(* Logix 5000 AddOnInstructionDefinition export Banner_QM30VT3_PD_v5; software revision 33.00 *)

TYPE Banner_QM30VT3_FP_RMS_PD_v5 :
STRUCT
   X_RMS_Velocity : REAL;   // in/sec or mm/sec
   Y_RMS_Velocity : REAL;   // in/sec or mm/sec
   Z_RMS_Velocity : REAL;   // in/sec or mm/sec
   X_High_Freq_RMS_Accel : REAL;   // G
   Y_High_Freq_RMS_Accel : REAL;   // G
   Z_High_Freq_RMS_Accel : REAL;   // G
   Temperature : REAL;   // F or C
   X : Banner_QM30VT3_FP_RMS_XYZ_PD_v5;
   Y : Banner_QM30VT3_FP_RMS_XYZ_PD_v5;
   Z : Banner_QM30VT3_FP_RMS_XYZ_PD_v5;
   Temp_Warning : BOOL;
   Temp_Alarm : BOOL;
END_STRUCT
END_TYPE

TYPE Banner_QM30VT3_FP_RMS_XYZ_PD_v5 :
STRUCT
   Vel_Acute_Warning : BOOL;
   Vel_Acute_Alarm : BOOL;
   Vel_Chronic_Warning : BOOL;
   Vel_Chronic_Alarm : BOOL;
   HiFreq_Accel_Acute_Warning : BOOL;
   HiFreq_Accel_Acute_Alarm : BOOL;
   HiFreq_Accel_Chronic_Warning : BOOL;
   HiFreq_Accel_Chronic_Alarm : BOOL;
END_STRUCT
END_TYPE

TYPE Banner_QM30VT3_PDI_v5 :
STRUCT
   PD0_FP_imperial : Banner_QM30VT3_FP_RMS_PD_v5;
   PD1_SS_imperial : Banner_QM30VT3_SS_RMS_PD_v5;
   PD2_FP_metric : Banner_QM30VT3_FP_RMS_PD_v5;
   PD3_SS_metric : Banner_QM30VT3_SS_RMS_PD_v5;
   PD4_User_metric : Banner_QM30VT3_User_PD_v5;
   PD5_User_imperial : Banner_QM30VT3_User_PD_v5;
   DTI : SINT[32];
END_STRUCT
END_TYPE

TYPE Banner_QM30VT3_SS_RMS_PD_HiFreq_v5 :
STRUCT
   High_Frequency_RMS_Accel : DINT;
   Scale : INT;
   HiFreq_Accel_Acute_Warning : BOOL;
   HiFreq_Accel_Acute_Alarm : BOOL;
   HiFreq_Accel_Chronic_Warning : BOOL;
   HiFreq_Accel_Chronice_Alarm : BOOL;
END_STRUCT
END_TYPE

TYPE Banner_QM30VT3_SS_RMS_PD_v5 :
STRUCT
   X_Velocity : Banner_QM30VT3_SS_RMS_Vel_PD_v5;
   Y_Velocity : Banner_QM30VT3_SS_RMS_Vel_PD_v5;
   Z_Velocity : Banner_QM30VT3_SS_RMS_Vel_PD_v5;
   X_HiFreq : Banner_QM30VT3_SS_RMS_PD_HiFreq_v5;
   Y_HiFreq : Banner_QM30VT3_SS_RMS_PD_HiFreq_v5;
   Z_HiFreq : Banner_QM30VT3_SS_RMS_PD_HiFreq_v5;
   Temperature : DINT;   // F or C
   Scale : INT;
   Temp_Warning : BOOL;
   Temp_Alarm : BOOL;
END_STRUCT
END_TYPE

TYPE Banner_QM30VT3_SS_RMS_Vel_PD_v5 :
STRUCT
   RMS_Velocity : DINT;   // in/s or mm/sec
   Scale : INT;
   Vel_Acute_Warning : BOOL;
   Vel_Acute_Alarm : BOOL;
   Vel_Chronic_Warning : BOOL;
   Vel_Chronic_Alarm : BOOL;
END_STRUCT
END_TYPE

TYPE Banner_QM30VT3_User_PD_v5 :
STRUCT
   Metric : REAL[8];
   M1_Chan_1_Warning : BOOL;
   M1_Chan_2_Alarm : BOOL;
   M2_Chan_1_Warning : BOOL;
   M2_Chan_2_Alarm : BOOL;
   M3_Chan_1_Warning : BOOL;
   M3_Chan_2_Alarm : BOOL;
   M4_Chan_1_Warning : BOOL;
   M4_Chan_2_Alarm : BOOL;
   M5_Chan_1_Warning : BOOL;
   M5_Chan_2_Alarm : BOOL;
   M6_Chan_1_Warning : BOOL;
   M6_Chan_2_Alarm : BOOL;
   M7_Chan_1_Warning : BOOL;
   M7_Chan_2_Alarm : BOOL;
END_STRUCT
END_TYPE

ADD_ON_INSTRUCTION Banner_QM30VT3_PD_FP_RMS_v5   (* revision 1.0 *)
VAR_IN_OUT
   Bytes : SINT[32]; {required}
   Data : Banner_QM30VT3_FP_RMS_PD_v5; {required}
END_VAR
VAR
   Temp : DINT[16]; {access None}
END_VAR

ROUTINE Logic   (* ladder *)
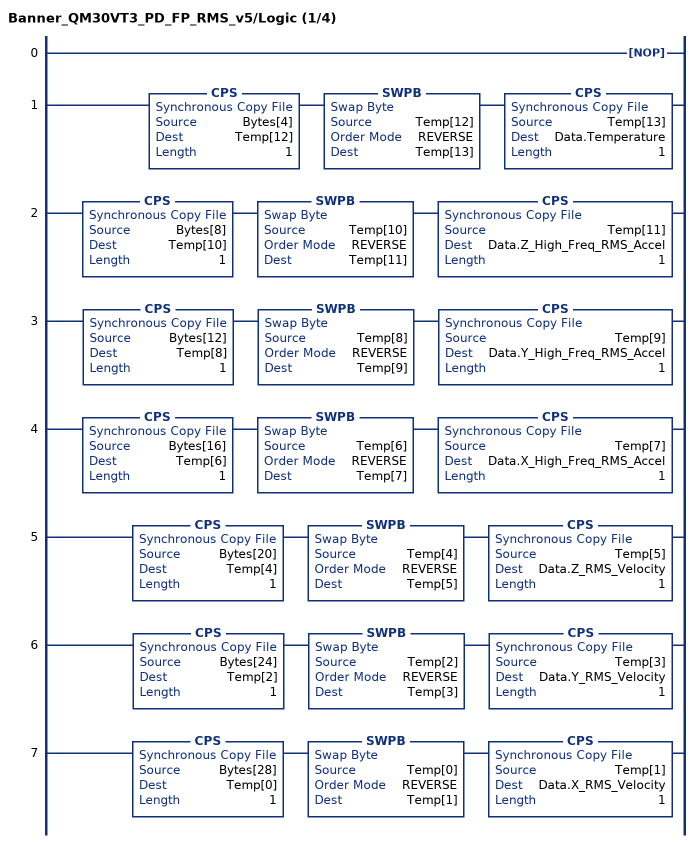
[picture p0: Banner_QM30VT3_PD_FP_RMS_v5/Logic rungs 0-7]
   0: NOP();
   1: CPS(Bytes[4],Temp[12],1)SWPB(Temp[12],REVERSE,Temp[13])CPS(Temp[13],Data.Temperature,1);
   2: CPS(Bytes[8],Temp[10],1)SWPB(Temp[10],REVERSE,Temp[11])CPS(Temp[11],Data.Z_High_Freq_RMS_Accel,1);
   3: CPS(Bytes[12],Temp[8],1)SWPB(Temp[8],REVERSE,Temp[9])CPS(Temp[9],Data.Y_High_Freq_RMS_Accel,1);
   4: CPS(Bytes[16],Temp[6],1)SWPB(Temp[6],REVERSE,Temp[7])CPS(Temp[7],Data.X_High_Freq_RMS_Accel,1);
   5: CPS(Bytes[20],Temp[4],1)SWPB(Temp[4],REVERSE,Temp[5])CPS(Temp[5],Data.Z_RMS_Velocity,1);
   6: CPS(Bytes[24],Temp[2],1)SWPB(Temp[2],REVERSE,Temp[3])CPS(Temp[3],Data.Y_RMS_Velocity,1);
   7: CPS(Bytes[28],Temp[0],1)SWPB(Temp[0],REVERSE,Temp[1])CPS(Temp[1],Data.X_RMS_Velocity,1);
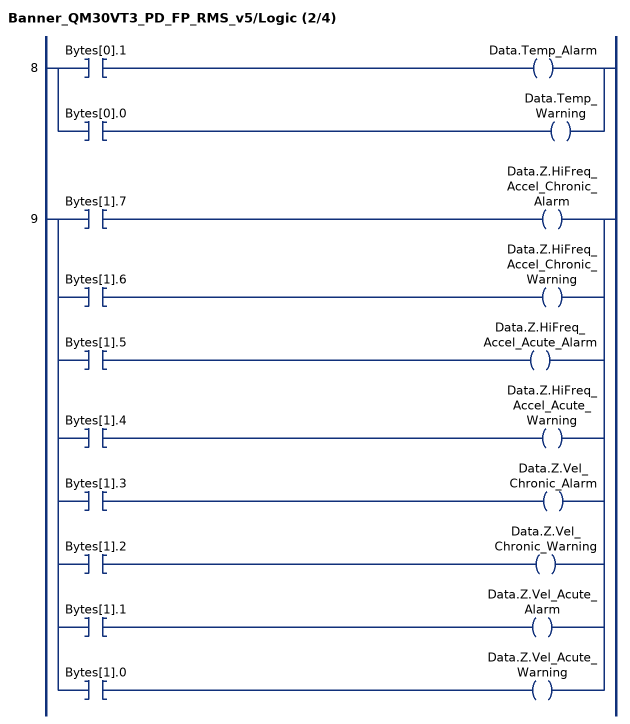
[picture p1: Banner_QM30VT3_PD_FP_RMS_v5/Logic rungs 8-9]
   8: [XIC(Bytes[0].1) OTE(Data.Temp_Alarm) ,XIC(Bytes[0].0) OTE(Data.Temp_Warning) ];
   9: [XIC(Bytes[1].7) OTE(Data.Z.HiFreq_Accel_Chronic_Alarm) ,XIC(Bytes[1].6) OTE(Data.Z.HiFreq_Accel_Chronic_Warning) ,XIC(Bytes[1].5) OTE(Data.Z.HiFreq_Accel_Acute_Alarm) ,XIC(Bytes[1].4) OTE(Data.Z.HiFreq_Accel_Acute_Warning) ,XIC(Bytes[1].3) OTE(Data.Z.Vel_Chronic_Alarm) ,XIC(Bytes[1].2) OTE(Data.Z.Vel_Chronic_Warning) ,XIC(Bytes[1].1) OTE(Data.Z.Vel_Acute_Alarm) ,XIC(Bytes[1].0) OTE(Data.Z.Vel_Acute_Warning) ];
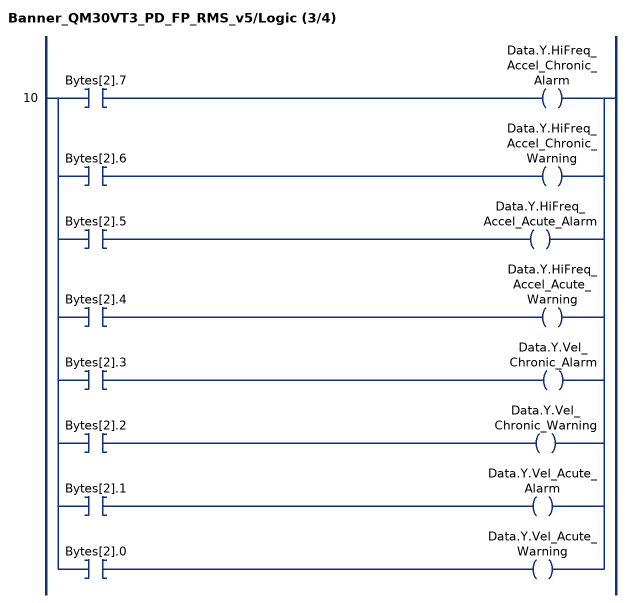
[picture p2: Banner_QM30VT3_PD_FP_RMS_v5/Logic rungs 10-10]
   10: [XIC(Bytes[2].7) OTE(Data.Y.HiFreq_Accel_Chronic_Alarm) ,XIC(Bytes[2].6) OTE(Data.Y.HiFreq_Accel_Chronic_Warning) ,XIC(Bytes[2].5) OTE(Data.Y.HiFreq_Accel_Acute_Alarm) ,XIC(Bytes[2].4) OTE(Data.Y.HiFreq_Accel_Acute_Warning) ,XIC(Bytes[2].3) OTE(Data.Y.Vel_Chronic_Alarm) ,XIC(Bytes[2].2) OTE(Data.Y.Vel_Chronic_Warning) ,XIC(Bytes[2].1) OTE(Data.Y.Vel_Acute_Alarm) ,XIC(Bytes[2].0) OTE(Data.Y.Vel_Acute_Warning) ];
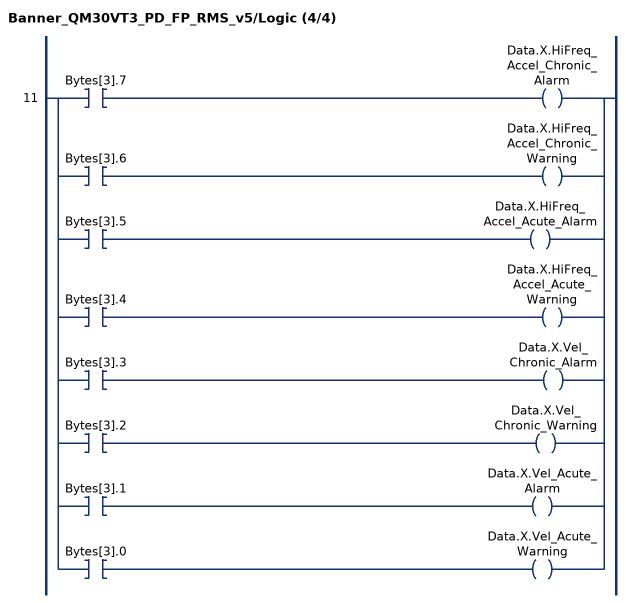
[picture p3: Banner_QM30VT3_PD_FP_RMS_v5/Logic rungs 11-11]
   11: [XIC(Bytes[3].7) OTE(Data.X.HiFreq_Accel_Chronic_Alarm) ,XIC(Bytes[3].6) OTE(Data.X.HiFreq_Accel_Chronic_Warning) ,XIC(Bytes[3].5) OTE(Data.X.HiFreq_Accel_Acute_Alarm) ,XIC(Bytes[3].4) OTE(Data.X.HiFreq_Accel_Acute_Warning) ,XIC(Bytes[3].3) OTE(Data.X.Vel_Chronic_Alarm) ,XIC(Bytes[3].2) OTE(Data.X.Vel_Chronic_Warning) ,XIC(Bytes[3].1) OTE(Data.X.Vel_Acute_Alarm) ,XIC(Bytes[3].0) OTE(Data.X.Vel_Acute_Warning) ];
END_ROUTINE
END_ADD_ON_INSTRUCTION

ADD_ON_INSTRUCTION Banner_QM30VT3_PD_SS_RMS_v5   (* revision 1.0 *)
VAR_IN_OUT
   Bytes : SINT[32]; {required}
   Data : Banner_QM30VT3_SS_RMS_PD_v5; {required}
END_VAR
VAR
   Temp : DINT[16]; {access None}
END_VAR

ROUTINE Logic   (* ladder *)
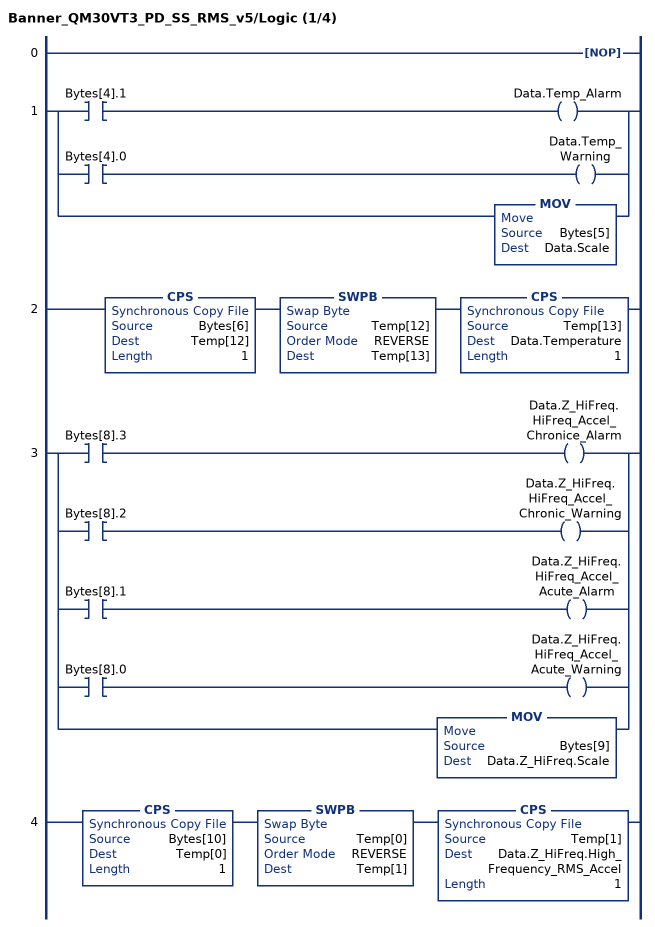
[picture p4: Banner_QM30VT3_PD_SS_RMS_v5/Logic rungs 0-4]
   0: NOP();
   1: [XIC(Bytes[4].1) OTE(Data.Temp_Alarm) ,XIC(Bytes[4].0) OTE(Data.Temp_Warning) ,MOV(Bytes[5],Data.Scale) ];
   2: CPS(Bytes[6],Temp[12],1)SWPB(Temp[12],REVERSE,Temp[13])CPS(Temp[13],Data.Temperature,1);
   3: [XIC(Bytes[8].3) OTE(Data.Z_HiFreq.HiFreq_Accel_Chronice_Alarm) ,XIC(Bytes[8].2) OTE(Data.Z_HiFreq.HiFreq_Accel_Chronic_Warning) ,XIC(Bytes[8].1) OTE(Data.Z_HiFreq.HiFreq_Accel_Acute_Alarm) ,XIC(Bytes[8].0) OTE(Data.Z_HiFreq.HiFreq_Accel_Acute_Warning) ,MOV(Bytes[9],Data.Z_HiFreq.Scale) ];
   4: CPS(Bytes[10],Temp[0],1)SWPB(Temp[0],REVERSE,Temp[1])CPS(Temp[1],Data.Z_HiFreq.High_Frequency_RMS_Accel,1);
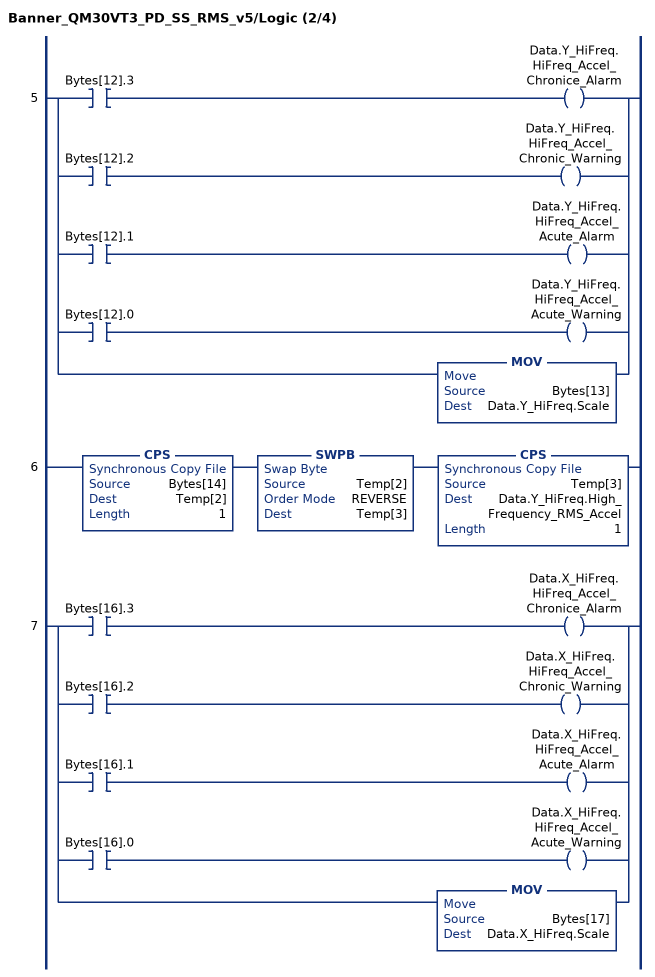
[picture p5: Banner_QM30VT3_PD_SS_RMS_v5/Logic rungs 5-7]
   5: [XIC(Bytes[12].3) OTE(Data.Y_HiFreq.HiFreq_Accel_Chronice_Alarm) ,XIC(Bytes[12].2) OTE(Data.Y_HiFreq.HiFreq_Accel_Chronic_Warning) ,XIC(Bytes[12].1) OTE(Data.Y_HiFreq.HiFreq_Accel_Acute_Alarm) ,XIC(Bytes[12].0) OTE(Data.Y_HiFreq.HiFreq_Accel_Acute_Warning) ,MOV(Bytes[13],Data.Y_HiFreq.Scale) ];
   6: CPS(Bytes[14],Temp[2],1)SWPB(Temp[2],REVERSE,Temp[3])CPS(Temp[3],Data.Y_HiFreq.High_Frequency_RMS_Accel,1);
   7: [XIC(Bytes[16].3) OTE(Data.X_HiFreq.HiFreq_Accel_Chronice_Alarm) ,XIC(Bytes[16].2) OTE(Data.X_HiFreq.HiFreq_Accel_Chronic_Warning) ,XIC(Bytes[16].1) OTE(Data.X_HiFreq.HiFreq_Accel_Acute_Alarm) ,XIC(Bytes[16].0) OTE(Data.X_HiFreq.HiFreq_Accel_Acute_Warning) ,MOV(Bytes[17],Data.X_HiFreq.Scale) ];
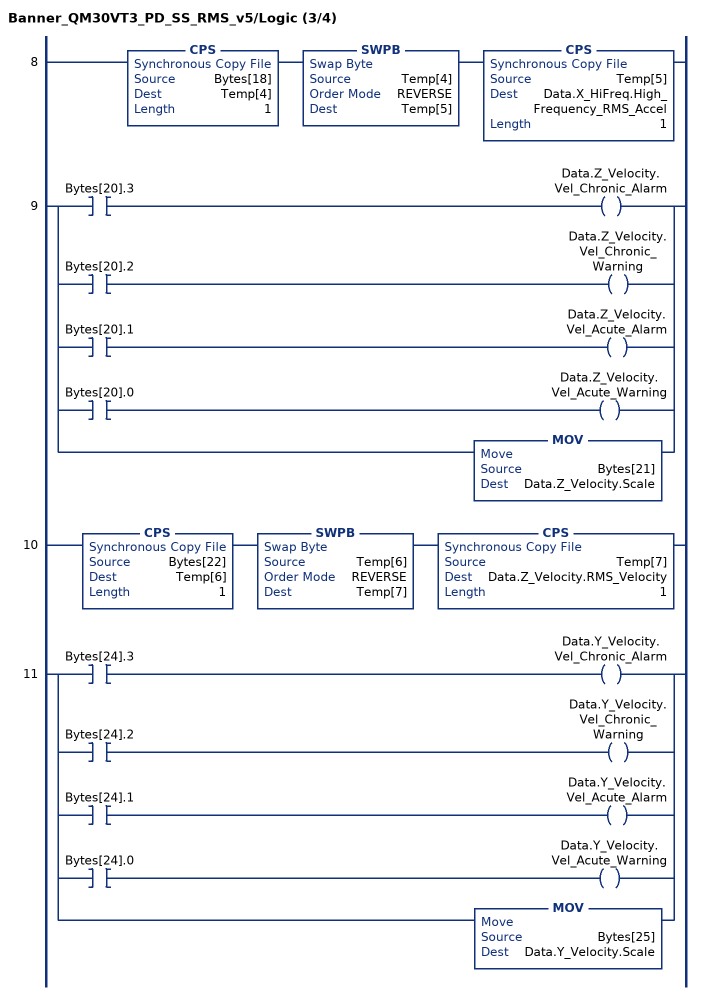
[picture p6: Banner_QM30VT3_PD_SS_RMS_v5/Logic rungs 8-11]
   8: CPS(Bytes[18],Temp[4],1)SWPB(Temp[4],REVERSE,Temp[5])CPS(Temp[5],Data.X_HiFreq.High_Frequency_RMS_Accel,1);
   9: [XIC(Bytes[20].3) OTE(Data.Z_Velocity.Vel_Chronic_Alarm) ,XIC(Bytes[20].2) OTE(Data.Z_Velocity.Vel_Chronic_Warning) ,XIC(Bytes[20].1) OTE(Data.Z_Velocity.Vel_Acute_Alarm) ,XIC(Bytes[20].0) OTE(Data.Z_Velocity.Vel_Acute_Warning) ,MOV(Bytes[21],Data.Z_Velocity.Scale) ];
   10: CPS(Bytes[22],Temp[6],1)SWPB(Temp[6],REVERSE,Temp[7])CPS(Temp[7],Data.Z_Velocity.RMS_Velocity,1);
   11: [XIC(Bytes[24].3) OTE(Data.Y_Velocity.Vel_Chronic_Alarm) ,XIC(Bytes[24].2) OTE(Data.Y_Velocity.Vel_Chronic_Warning) ,XIC(Bytes[24].1) OTE(Data.Y_Velocity.Vel_Acute_Alarm) ,XIC(Bytes[24].0) OTE(Data.Y_Velocity.Vel_Acute_Warning) ,MOV(Bytes[25],Data.Y_Velocity.Scale) ];
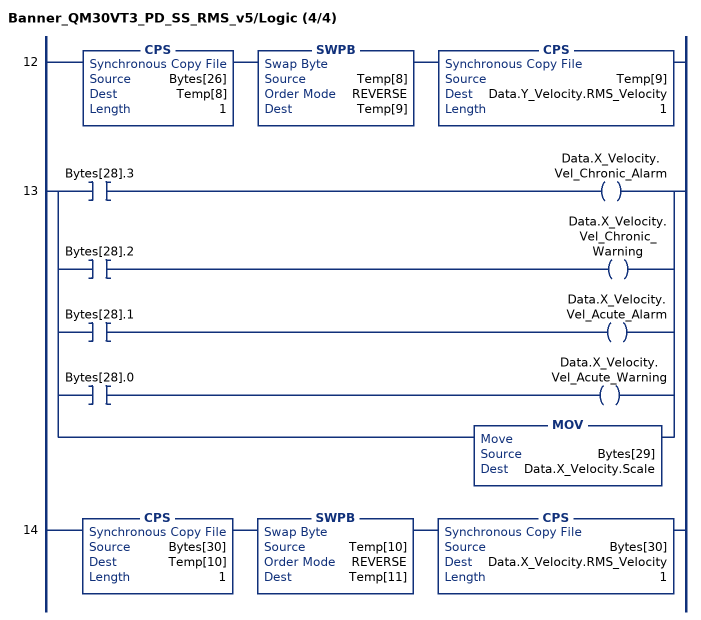
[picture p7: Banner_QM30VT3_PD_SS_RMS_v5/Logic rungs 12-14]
   12: CPS(Bytes[26],Temp[8],1)SWPB(Temp[8],REVERSE,Temp[9])CPS(Temp[9],Data.Y_Velocity.RMS_Velocity,1);
   13: [XIC(Bytes[28].3) OTE(Data.X_Velocity.Vel_Chronic_Alarm) ,XIC(Bytes[28].2) OTE(Data.X_Velocity.Vel_Chronic_Warning) ,XIC(Bytes[28].1) OTE(Data.X_Velocity.Vel_Acute_Alarm) ,XIC(Bytes[28].0) OTE(Data.X_Velocity.Vel_Acute_Warning) ,MOV(Bytes[29],Data.X_Velocity.Scale) ];
   14: CPS(Bytes[30],Temp[10],1)SWPB(Temp[10],REVERSE,Temp[11])CPS(Bytes[30],Data.X_Velocity.RMS_Velocity,1);
END_ROUTINE
END_ADD_ON_INSTRUCTION

ADD_ON_INSTRUCTION Banner_QM30VT3_PD_User_v5   (* revision 1.0 *)
VAR_IN_OUT
   Bytes : SINT[32]; {required}
   Data : Banner_QM30VT3_User_PD_v5; {required}
END_VAR
VAR
   Temp : DINT[16]; {access None}
END_VAR

ROUTINE Logic   (* ladder *)
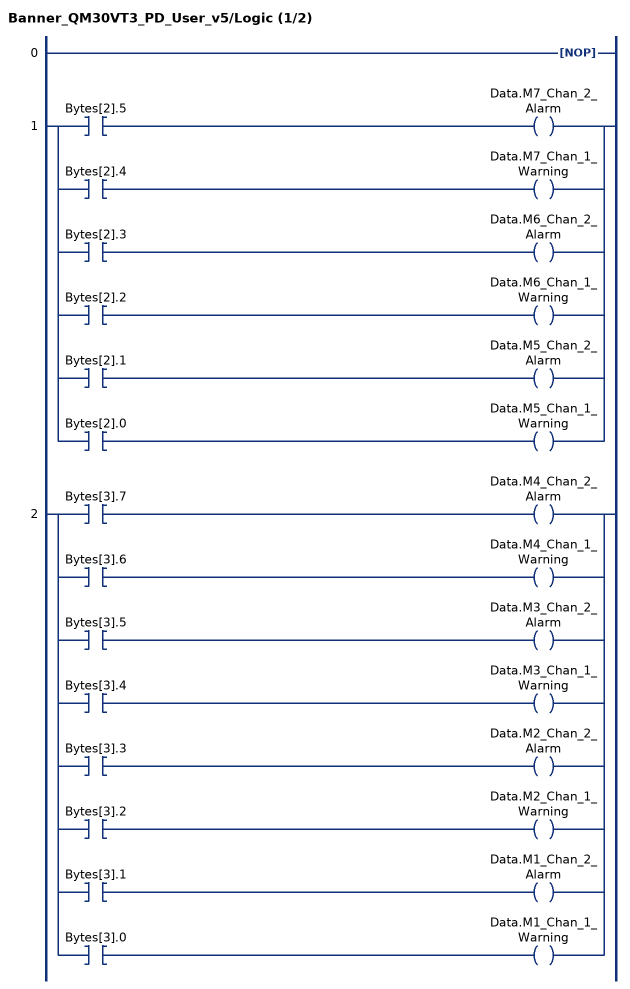
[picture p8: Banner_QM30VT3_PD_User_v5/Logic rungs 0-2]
   0: NOP();
   1: [XIC(Bytes[2].5) OTE(Data.M7_Chan_2_Alarm) ,XIC(Bytes[2].4) OTE(Data.M7_Chan_1_Warning) ,XIC(Bytes[2].3) OTE(Data.M6_Chan_2_Alarm) ,XIC(Bytes[2].2) OTE(Data.M6_Chan_1_Warning) ,XIC(Bytes[2].1) OTE(Data.M5_Chan_2_Alarm) ,XIC(Bytes[2].0) OTE(Data.M5_Chan_1_Warning) ];
   2: [XIC(Bytes[3].7) OTE(Data.M4_Chan_2_Alarm) ,XIC(Bytes[3].6) OTE(Data.M4_Chan_1_Warning) ,XIC(Bytes[3].5) OTE(Data.M3_Chan_2_Alarm) ,XIC(Bytes[3].4) OTE(Data.M3_Chan_1_Warning) ,XIC(Bytes[3].3) OTE(Data.M2_Chan_2_Alarm) ,XIC(Bytes[3].2) OTE(Data.M2_Chan_1_Warning) ,XIC(Bytes[3].1) OTE(Data.M1_Chan_2_Alarm) ,XIC(Bytes[3].0) OTE(Data.M1_Chan_1_Warning) ];
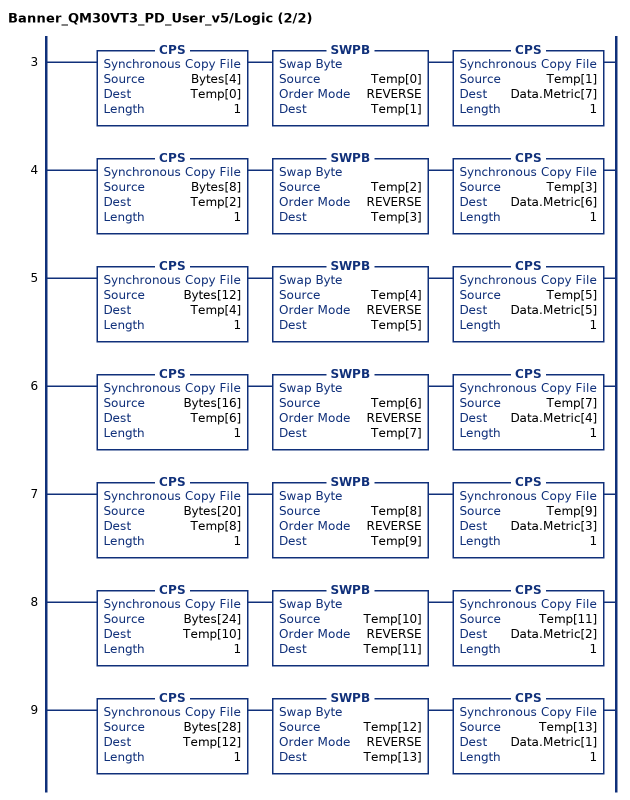
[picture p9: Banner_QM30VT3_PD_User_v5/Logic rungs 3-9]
   3: CPS(Bytes[4],Temp[0],1)SWPB(Temp[0],REVERSE,Temp[1])CPS(Temp[1],Data.Metric[7],1);
   4: CPS(Bytes[8],Temp[2],1)SWPB(Temp[2],REVERSE,Temp[3])CPS(Temp[3],Data.Metric[6],1);
   5: CPS(Bytes[12],Temp[4],1)SWPB(Temp[4],REVERSE,Temp[5])CPS(Temp[5],Data.Metric[5],1);
   6: CPS(Bytes[16],Temp[6],1)SWPB(Temp[6],REVERSE,Temp[7])CPS(Temp[7],Data.Metric[4],1);
   7: CPS(Bytes[20],Temp[8],1)SWPB(Temp[8],REVERSE,Temp[9])CPS(Temp[9],Data.Metric[3],1);
   8: CPS(Bytes[24],Temp[10],1)SWPB(Temp[10],REVERSE,Temp[11])CPS(Temp[11],Data.Metric[2],1);
   9: CPS(Bytes[28],Temp[12],1)SWPB(Temp[12],REVERSE,Temp[13])CPS(Temp[13],Data.Metric[1],1);
END_ROUTINE
END_ADD_ON_INSTRUCTION

ADD_ON_INSTRUCTION Banner_QM30VT3_PD_v5   (* revision 5.0 *)
VAR_IN_OUT
   QM30VT3 : Banner_QM30VT3_PDI_v5; {required}
END_VAR
VAR_INPUT
   Configuration : DINT; {required}
   Byte_Swap : BOOL; {required}
END_VAR
VAR
   Status_FP_RMS : Banner_QM30VT3_PD_FP_RMS_v5[2]; {access None}
   Status_SS_RMS : Banner_QM30VT3_PD_SS_RMS_v5[2]; {access None}
   Status_User : Banner_QM30VT3_PD_User_v5[2]; {access None}
END_VAR

ROUTINE Logic   (* ladder *)
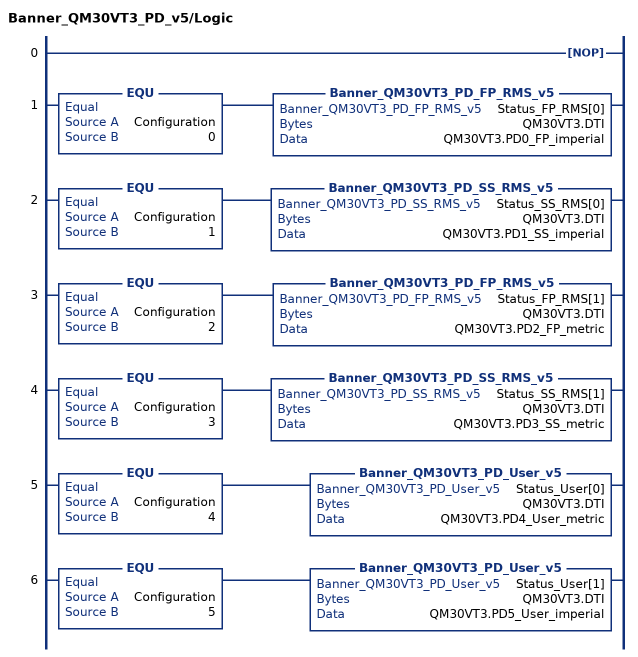
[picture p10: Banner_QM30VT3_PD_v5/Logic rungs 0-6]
   0: NOP();
   1: EQU(Configuration,0)Banner_QM30VT3_PD_FP_RMS_v5(Status_FP_RMS[0],QM30VT3.DTI,QM30VT3.PD0_FP_imperial);
   2: EQU(Configuration,1)Banner_QM30VT3_PD_SS_RMS_v5(Status_SS_RMS[0],QM30VT3.DTI,QM30VT3.PD1_SS_imperial);
   3: EQU(Configuration,2)Banner_QM30VT3_PD_FP_RMS_v5(Status_FP_RMS[1],QM30VT3.DTI,QM30VT3.PD2_FP_metric);
   4: EQU(Configuration,3)Banner_QM30VT3_PD_SS_RMS_v5(Status_SS_RMS[1],QM30VT3.DTI,QM30VT3.PD3_SS_metric);
   5: EQU(Configuration,4)Banner_QM30VT3_PD_User_v5(Status_User[0],QM30VT3.DTI,QM30VT3.PD4_User_metric);
   6: EQU(Configuration,5)Banner_QM30VT3_PD_User_v5(Status_User[1],QM30VT3.DTI,QM30VT3.PD5_User_imperial);
END_ROUTINE
END_ADD_ON_INSTRUCTION
